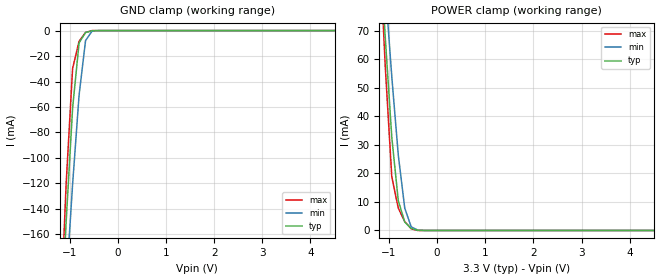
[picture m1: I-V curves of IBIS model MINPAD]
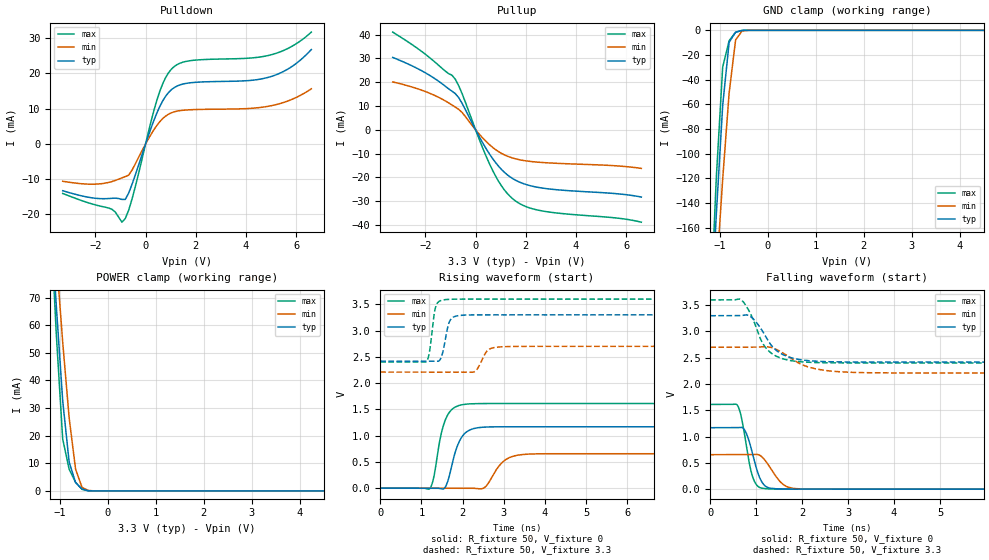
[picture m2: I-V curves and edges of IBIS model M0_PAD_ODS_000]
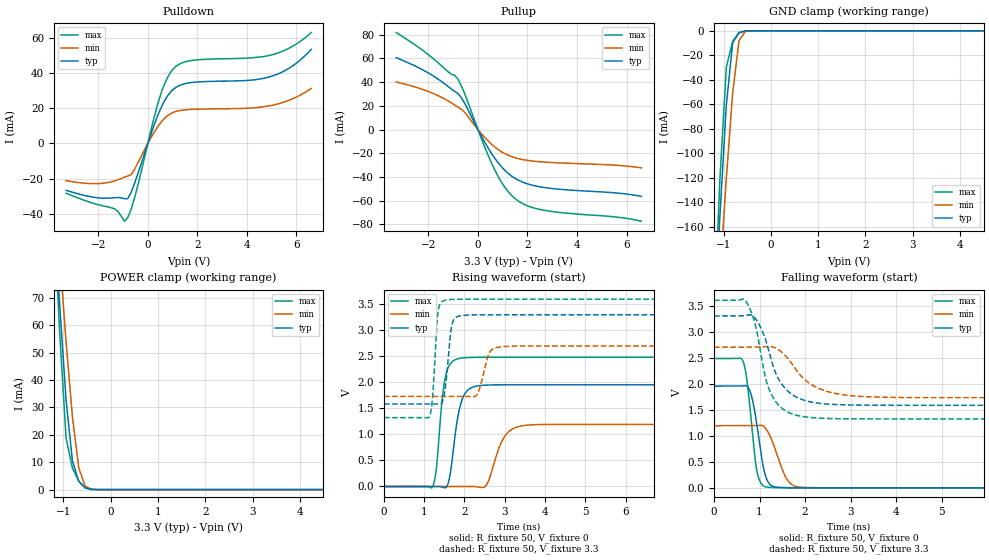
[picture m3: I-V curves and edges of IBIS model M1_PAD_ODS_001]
|   Microsemi Corporation
|   SmartFusion2 Automotive IBIS Model
[IBIS ver]   5.0
[File name]   as30208cg_33v_rev1p1.ibs
[File Rev]   1.1
[Date]   Wed Apr 02 2025
[Source] Simulated Models ONLY.
   All data is based on Spice simulation. All performed at Microsemi Corporation.
   Please refer to the Microsemi website for future updates at www.microsemi.com
[Notes]  Microsemi SmartFusion2 IBIS models for automotive operating conditions
   for DDRIO IO Banks IO Configurations ONLY. Models uses a software default
   fixed codes except for DDR3/SSTL15 which will always require calibrated
   codes.
   Automotive Temperature Grade 2 (t2) models cover a temperature range from
   -40C to 125C.
   Please refer to msio_auto_t2.ibs for MSIO IO Banks IO Configurations.
   Please refer to msiod_auto_t2.ibs for MSIOD IO Banks IO Configurations.
   The package parasitics of various package types are given.
   Uncomment the appropriate package or refer to the .pkg for specific
   per pin parasitic data.
   There are warnings related to non-monotonic and Increasing/Decreasing Current.
   They are expected on 20 Ohms and 30 Ohms I/O ODT models in DDR3/SSTL15.
[Disclaimer] This information is for board design considerations.
   Simulation based V/I curves contained in this model file are
   considered preliminary until verified against bench
   measurements. Maximum currents may vary from part to part but
   should not exceed maximum I/V curves provided in this model file.
[Copyright]  (c) 2015, Microsemi Corporation, All Rights Reserved.
| IBIS MODEL CHECKLIST
| Microsemi is dedicated to releasing quality IBIS models to customers.
| The following items have been
| verified for this IBIS model before release:
| 1)  Checked IBIS model by the golden parser ibischk5 [Complete]
| 2)  Ensured no errors reported by golden parser
|   for the IBIS model [Complete]
| 3)  Defined Vinl and Vinh for recievers [Complete]
| 4)  Defined Standard Load and Vmeas values for drivers [Complete]
| 5)  Defined overshoots for drivers and recievers [NA]
| 6)  Validated Ramp Values[Complete]
| 7)  Defined V-T Tables for all output drivers [Complete]
| 8)  Validated [Diff Pins] []
| 9)  Verified Package Parasitics [Complete]
| 10) Defined Standard Load Parameters and Specifications
|   for waveforms [Complete]
| 11) Defined and Validate Pin mappings [Complete]
| 12) Verified Ccomp Value []
| 13) Visually Inspected I-V Curves and V-T Tables  [Complete]
| 14) Presented Typ/Min/Max Values in the correct order for
|   all tables and parameters [Complete]
| 15) Simulated all output models with standard load and
|   switching through Vmeas [Complete]
| 16) Simulated all reciever models  [Complete]
| 17) Validated Models selectors. []
| 18) Visually inspected Spice and IBIS correlation for
|   a) Typical VT Curves [Complete]
|   b) Minimum VT Curves [Complete]
|   c) Maximum VT Curves [Complete]
| 19) Visually inspected Silicon and IBIS correlation
|   a) Typical IV Pull UP/ Pull Down Curves []
|   b) Minimum IV Pull UP/ Pull Down Curves []
|   c) Maximum IV Pull UP/ Pull Down Curves []
|   Component SmartFusion2
[Component]   SmartFusion2 W MRAM
[Manufacturer]   Avalanche Technology
[Package]
|  Design die-package: BGA
| variable   typ   min   max
R_pkg   0.72029   0.51528   1.0002
L_pkg   5.797e-9   4.155e-9   8.073e-9
C_pkg   1.116e-12   7.907e-13   1.753e-12
|Pin and Model info
[Pin]  signal_name  model_name   R_pin   L_pin   C_pin
L9   CS1#   MINPAD   0.4340		15.2000E-9		1.2600E-12
J10   CS2#   MINPAD   0.3800		13.5000E-9		1.0400E-12
K9   CLK1   MINPAD   0.4300		12.7000E-9		0.9790E-12
K8   CLK2   MINPAD   0.4480		14.6000E-9		1.1600E-12
M10   IO_0   MIOPAD   0.4010		12.4000E-9		1.2500E-12
M9   IO_1   MIOPAD   0.4050		14.2000E-9		1.1100E-12
L11   IO_2   MIOPAD   0.3780		11.8000E-9		1.2000E-12
M11   IO_3   MIOPAD   0.3700		11.8000E-9		1.2600E-12
M12   IO_4   MIOPAD   0.3710		11.1000E-9		1.1000E-12
N10   IO_5   MIOPAD   0.4050		13.8000E-9		1.1600E-12
N9   IO_6   MIOPAD   0.3830		15.2000E-9		1.0900E-12
N8   IO_7   MIOPAD   0.4480		16.4000E-9		1.0800E-12
J14   HTBSEL   MINPAD   0.1380		6.1700E-9		0.6060E-12
H14   HBP_2   MINPAD   0.1470		6.3900E-9		1.0000E-12
G13   HBP_1   MINPAD   0.1910		8.5000E-9		1.1500E-12
G12   HBP_0   MINPAD   0.2050		8.6800E-9		1.4200E-12
J11   RESET#   MINPAD   0.3410		14.1000E-9		1.6300E-12
J12   INT1#   MIOPAD   0.3080		12.5000E-9		1.2100E-12
K10   INT2#   MIOPAD   0.2120		10.3000E-9		0.8230E-12
M7   VSSIO   GND   NA   NA   NA
H8   VSSIO   GND   NA   NA   NA
L8   VSSIO   GND   NA   NA   NA
P10   VSSIO   GND   NA   NA   NA
H12   VSSIO   GND   NA   NA   NA
N12   VSSIO   GND   NA   NA   NA
P12   VSSIO   GND   NA   NA   NA
H13   VSSIO   GND   NA   NA   NA
N13   VSSIO   GND   NA   NA   NA
A3   VSS   GND   NA   NA   NA
B3   VSS   GND   NA   NA   NA
W3   VSS   GND   NA   NA   NA
Y3   VSS   GND   NA   NA   NA
A4   VSS   GND   NA   NA   NA
Y4   VSS   GND   NA   NA   NA
F5   VSS   GND   NA   NA   NA
G5   VSS   GND   NA   NA   NA
P5   VSS   GND   NA   NA   NA
R5   VSS   GND   NA   NA   NA
F6   VSS   GND   NA   NA   NA
H6   VSS   GND   NA   NA   NA
J6   VSS   GND   NA   NA   NA
L6   VSS   GND   NA   NA   NA
N6   VSS   GND   NA   NA   NA
R6   VSS   GND   NA   NA   NA
L7   VSS   GND   NA   NA   NA
N7   VSS   GND   NA   NA   NA
G8   VSS   GND   NA   NA   NA
P8   VSS   GND   NA   NA   NA
G10   VSS   GND   NA   NA   NA
H10   VSS   GND   NA   NA   NA
L12   VSS   GND   NA   NA   NA
L13   VSS   GND   NA   NA   NA
P13   VSS   GND   NA   NA   NA
F14   VSS   GND   NA   NA   NA
L14   VSS   GND   NA   NA   NA
N14   VSS   GND   NA   NA   NA
R14   VSS   GND   NA   NA   NA
F15   VSS   GND   NA   NA   NA
G15   VSS   GND   NA   NA   NA
P15   VSS   GND   NA   NA   NA
R15   VSS   GND   NA   NA   NA
A16   VSS   GND   NA   NA   NA
Y16   VSS   GND   NA   NA   NA
A17   VSS   GND   NA   NA   NA
B17   VSS   GND   NA   NA   NA
W17   VSS   GND   NA   NA   NA
Y17   VSS   GND   NA   NA   NA
G6   VCCIO   POWER   NA   NA   NA
P6   VCCIO   POWER   NA   NA   NA
G7   VCCIO   POWER   NA   NA   NA
J7   VCCIO   POWER   NA   NA   NA
P7   VCCIO   POWER   NA   NA   NA
M8   VCCIO   POWER   NA   NA   NA
H9   VCCIO   POWER   NA   NA   NA
H11   VCCIO   POWER   NA   NA   NA
N11   VCCIO   POWER   NA   NA   NA
J13   VCCIO   POWER   NA   NA   NA
M13   VCCIO   POWER   NA   NA   NA
G14   VCCIO   POWER   NA   NA   NA
P14   VCCIO   POWER   NA   NA   NA
K6   VCC   POWER   NA   NA   NA
M6   VCC   POWER   NA   NA   NA
K7   VCC   POWER   NA   NA   NA
G9   VCC   POWER   NA   NA   NA
P9   VCC   POWER   NA   NA   NA
G11   VCC   POWER   NA   NA   NA
K11   VCC   POWER   NA   NA   NA
P11   VCC   POWER   NA   NA   NA
K13   VCC   POWER   NA   NA   NA
K14   VCC   POWER   NA   NA   NA
M14   VCC   POWER   NA   NA   NA
K12   VDD   POWER   NA   NA   NA
| END PIN INFO
| IOPAD
[Model Selector] MIOPAD
| Model Description
M0_PAD_ODS_000   ODS_000
M1_PAD_ODS_001   ODS_001
M2_PAD_ODS_010   ODS_010
M3_PAD_ODS_011   ODS_011
M4_PAD_ODS_100   ODS_100
M5_PAD_ODS_101   ODS_101
M6_PAD_ODS_110   ODS_110
M7_PAD_ODS_111   ODS_111
| Models and submodels in the file (9): MINPAD (Input), M0_PAD_ODS_000 (I/O), M1_PAD_ODS_001 (I/O), M2_PAD_ODS_010 (I/O), M3_PAD_ODS_011 (I/O), M4_PAD_ODS_100 (I/O), M5_PAD_ODS_101 (I/O), M6_PAD_ODS_110 (I/O), M7_PAD_ODS_111 (I/O)
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[Model] MINPAD
Model_type Input
Enable   Active-High
Vinl  =  0.8
Vinh  =  2.2
| Capacitance  typ   min   max
C_comp   1.514821e-12   1.418868e-12   1.647023e-12
| Variables   typ   min   max
[GND Clamp Reference]   0   0   0
[POWER Clamp Reference]   3.3   2.7   3.6
[Pulldown Reference]   0   0   0
[Pullup Reference]   3.3   2.7   3.6
[Temperature Range]   25   125   -40
[Voltage Range]   3.3   2.7   3.6
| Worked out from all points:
|   GND clamp passes 1 mA (typ) near -0.62 V on its own axis
|   POWER clamp passes 1 mA (typ) near -0.56 V on its own axis
[GND Clamp]
| Voltage   I(typ)   I(min)   I(max)
-3.3V     -1.961A    -1.697A    -2.357A
-1.21V    -250.7mA   -283.7mA   -242.5mA
-1.076V   -150.6mA   -200.1mA   -120.6mA
-941.4mV  -60.83mA   -120.8mA   -29.75mA
-806.9mV  -9.646mA   -50.71mA   -8.435mA
-672.4mV  -1.585mA   -7.866mA   -1.457mA
-537.9mV  -71.75uA   -504.3uA   -18.73uA
-403.4mV  -593.9nA   -18.57uA   -37.22nA
6.6V      0A         0A         0A
[POWER Clamp]
| Voltage   I(typ)   I(min)   I(max)
-3.3V     772.3mA    673.3mA    930.5mA
-1.21V    105.9mA    117.6mA    104.6mA
-1.076V   67.34mA    85.06mA    57.16mA
-941.4mV  32.71mA    53.93mA    18.82mA
-806.9mV  10.48mA    26.53mA    7.848mA
-672.4mV  2.975mA    7.856mA    3.108mA
-537.9mV  710.9uA    1.248mA    573.1uA
-403.4mV  60.69uA    160.8uA    9.187uA
-269mV    142.4nA    6.118uA    23.26nA
6.6V      0A         0A         0A
[Model] M0_PAD_ODS_000
Model_type I/O
Enable   Active-High
Vinl  =  0.8
Vinh  =  2.2
Vmeas =  1.65
Cref  =  30e-12
| Capacitance  typ   min   max
C_comp   1.518749e-12   1.424706e-12   1.652746e-12
| Variables   typ   min   max
[GND Clamp Reference]   0   0   0
[POWER Clamp Reference]   3.3   2.7   3.6
[Pulldown Reference]   0   0   0
[Pullup Reference]   3.3   2.7   3.6
[Temperature Range]   25   125   -40
[Voltage Range]   3.3   2.7   3.6
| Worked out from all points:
|   slope of the pulldown table from 0 to 0.495 V, typ, clamps not added: 52.1 ohm
|   slope of the pullup table from 0 to 0.495 V, typ, clamps not added: 53.8 ohm
|   GND clamp passes 1 mA (typ) near -0.62 V on its own axis
|   POWER clamp passes 1 mA (typ) near -0.56 V on its own axis
|   falling waveform, R_fixture 50, V_fixture 0: 20-80 % time 230ps typ, 320ps min, 198ps max; typ from 1.17 V to 0 V
|   falling waveform, R_fixture 50, V_fixture 3.3: 20-80 % time 464ps typ, 644ps min, 396ps max; typ from 3.3 V to 2.42 V
|   rising waveform, R_fixture 50, V_fixture 0: 20-80 % time 273ps typ, 362ps min, 248ps max; typ from 0 V to 1.17 V
|   rising waveform, R_fixture 50, V_fixture 3.3: 20-80 % time 138ps typ, 198ps min, 114ps max; typ from 2.42 V to 3.3 V
[GND Clamp]
| Voltage   I(typ)   I(min)   I(max)
-3.3V     -1.961A    -1.697A    -2.357A
-1.21V    -250.7mA   -283.7mA   -242.5mA
-1.076V   -150.6mA   -200.1mA   -120.7mA
-941.4mV  -60.83mA   -120.8mA   -29.76mA
-806.9mV  -9.649mA   -50.71mA   -8.442mA
-672.4mV  -1.587mA   -7.866mA   -1.46mA
-537.9mV  -71.93uA   -504.3uA   -18.83uA
-403.4mV  -595.6nA   -18.58uA   -37.45nA
6.6V      0A         0A         0A
[POWER Clamp]
| Voltage   I(typ)   I(min)   I(max)
-3.3V     772.3mA    673.3mA    930.5mA
-1.21V    105.9mA    117.6mA    104.6mA
-1.076V   67.34mA    85.06mA    57.16mA
-941.4mV  32.71mA    53.93mA    18.82mA
-806.9mV  10.48mA    26.53mA    7.848mA
-672.4mV  2.975mA    7.856mA    3.108mA
-537.9mV  710.9uA    1.248mA    573.1uA
-403.4mV  60.69uA    160.8uA    9.187uA
-269mV    142.4nA    6.118uA    23.26nA
6.6V      0A         0A         0A
[Pulldown]
| Voltage   I(typ)   I(min)   I(max)
-3.3V     -13.26mA   -10.58mA   -14.05mA
-1.345V   -15.42mA   -10.67mA   -18.51mA
-941.4mV  -15.74mA   -9.611mA   -22.19mA
-806.9mV  -15.73mA   -9.263mA   -21.14mA
-537.9mV  -11.42mA   -7.417mA   -15.59mA
455.2mV   8.881mA    5.308mA    12.55mA
682.8mV   12.23mA    7.205mA    17.1mA
1.024V    15.38mA    8.837mA    21.2mA
1.821V    17.39mA    9.724mA    23.68mA
4.914V    18.96mA    10.73mA    25.16mA
5.783V    21.77mA    12.53mA    27.53mA
6.6V      26.8mA     15.66mA    31.75mA
[Pullup]
| Voltage   I(typ)   I(min)   I(max)
-3.3V     30.44mA    20.14mA    41.1mA
-1.883V   23.26mA    15.61mA    30.81mA
-806.9mV  15.23mA    9.539mA    21.27mA
-537.9mV  11.14mA    7.294mA    15.26mA
227.6mV   -4.448mA   -2.796mA   -6.209mA
682.8mV   -12.17mA   -7.42mA    -17.15mA
1.138V    -17.78mA   -10.49mA   -25.16mA
1.593V    -21.21mA   -12.21mA   -29.96mA
2.048V    -23.14mA   -13.13mA   -32.47mA
2.731V    -24.61mA   -13.8mA    -34.27mA
5.659V    -26.92mA   -15.2mA    -37.16mA
6.6V      -28.29mA   -16.23mA   -38.86mA
[Ramp]
dV/dt_r   0.701574/0.273396n  0.393696/0.362182n  0.967082/0.24767n
dV/dt_f   0.529393/0.463707n  0.294233/0.644316n  0.719379/0.396117n
R_load = 50
[Falling Waveform]
R_fixture = 50
V_fixture = 0
V_fixture_min = 0
V_fixture_max = 0
| Time   V(typ)   V(min)   V(max)
0s        1.169V     656.2mV    1.612V
592.6ps   1.17V      656.6mV    1.594V
662.7ps   1.175V     656.6mV    1.423V
757.8ps   1.11V      656.7mV    979.6mV
920.8ps   673.8mV    658.3mV    236.4mV
1.068ns   233.8mV    649.1mV    35.66mV
1.221ns   45.34mV    516.2mV    8.708mV
1.592ns   3.21mV     87.01mV    1.102mV
2.018ns   581.9uV    4.7mV      706uV
21.88ns   211nV      -2.279uV   3.818uV
[Falling Waveform]
R_fixture = 50
V_fixture = 3.3
V_fixture_min = 2.7
V_fixture_max = 3.6
| Time   V(typ)   V(min)   V(max)
0s        3.3V       2.7V       3.6V
662.6ps   3.302V     2.701V     3.609V
894.9ps   3.273V     2.701V     3.302V
1.117ns   3.036V     2.709V     2.815V
1.233ns   2.866V     2.709V     2.664V
1.51ns    2.594V     2.628V     2.502V
2.006ns   2.457V     2.366V     2.42V
2.5ns     2.427V     2.259V     2.405V
3.502ns   2.418V     2.214V     2.401V
21.88ns   2.418V     2.21V      2.401V
[Rising Waveform]
R_fixture = 50
V_fixture = 0
V_fixture_min = 0
V_fixture_max = 0
| Time   V(typ)   V(min)   V(max)
0s        11.89nV    88.47nV    -73.19nV
1.207ns   -862.4uV   -520.5uV   -4.427mV
1.285ns   -918.3uV   -554.2uV   157.9mV
1.593ns   39.36mV    -686.9uV   1.324V
1.858ns   773.7mV    -801.1uV   1.558V
2.069ns   1.055V     -892.4uV   1.599V
2.519ns   1.162V     5.17mV     1.611V
2.991ns   1.169V     510.2mV    1.611V
3.605ns   1.169V     648.6mV    1.611V
21.88ns   1.169V     656.2mV    1.612V
[Rising Waveform]
R_fixture = 50
V_fixture = 3.3
V_fixture_min = 2.7
V_fixture_max = 3.6
| Time   V(typ)   V(min)   V(max)
0s        2.418V     2.21V      2.401V
1.115ns   2.419V     2.21V      2.406V
1.19ns    2.419V     2.21V      2.571V
1.354ns   2.418V     2.21V      3.473V
1.494ns   2.522V     2.21V      3.578V
1.647ns   3.091V     2.21V      3.594V
2.284ns   3.299V     2.216V     3.599V
2.637ns   3.299V     2.641V     3.599V
3.102ns   3.299V     2.696V     3.599V
21.88ns   3.3V       2.7V       3.6V
[Model] M1_PAD_ODS_001
Model_type I/O
Enable   Active-High
Vinl  =  0.8
Vinh  =  2.2
Vmeas =  1.65
Cref  =  30e-12
| Capacitance  typ   min   max
C_comp   1.518749e-12   1.424706e-12   1.652746e-12
| Variables   typ   min   max
[GND Clamp Reference]   0   0   0
[POWER Clamp Reference]   3.3   2.7   3.6
[Pulldown Reference]   0   0   0
[Pullup Reference]   3.3   2.7   3.6
[Temperature Range]   25   125   -40
[Voltage Range]   3.3   2.7   3.6
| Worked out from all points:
|   slope of the pulldown table from 0 to 0.495 V, typ, clamps not added: 26.1 ohm
|   slope of the pullup table from 0 to 0.495 V, typ, clamps not added: 27 ohm
|   GND clamp passes 1 mA (typ) near -0.62 V on its own axis
|   POWER clamp passes 1 mA (typ) near -0.56 V on its own axis
|   falling waveform, R_fixture 50, V_fixture 0: 20-80 % time 211ps typ, 305ps min, 176ps max; typ from 1.95 V to 0 V
|   falling waveform, R_fixture 50, V_fixture 3.3: 20-80 % time 457ps typ, 660ps min, 366ps max; typ from 3.3 V to 1.58 V
|   rising waveform, R_fixture 50, V_fixture 0: 20-80 % time 225ps typ, 335ps min, 176ps max; typ from 0 V to 1.95 V
|   rising waveform, R_fixture 50, V_fixture 3.3: 20-80 % time 129ps typ, 193ps min, 104ps max; typ from 1.58 V to 3.3 V
[GND Clamp]
| Voltage   I(typ)   I(min)   I(max)
-3.3V     -1.961A    -1.697A    -2.357A
-1.21V    -250.7mA   -283.7mA   -242.5mA
-1.076V   -150.6mA   -200.1mA   -120.7mA
-941.4mV  -60.83mA   -120.8mA   -29.76mA
-806.9mV  -9.649mA   -50.71mA   -8.442mA
-672.4mV  -1.587mA   -7.866mA   -1.46mA
-537.9mV  -71.93uA   -504.3uA   -18.83uA
-403.4mV  -595.6nA   -18.58uA   -37.45nA
6.6V      0A         0A         0A
[POWER Clamp]
| Voltage   I(typ)   I(min)   I(max)
-3.3V     772.3mA    673.3mA    930.5mA
-1.21V    105.9mA    117.6mA    104.6mA
-1.076V   67.34mA    85.06mA    57.16mA
-941.4mV  32.71mA    53.93mA    18.82mA
-806.9mV  10.48mA    26.53mA    7.848mA
-672.4mV  2.975mA    7.856mA    3.108mA
-537.9mV  710.9uA    1.248mA    573.1uA
-403.4mV  60.69uA    160.8uA    9.187uA
-269mV    142.4nA    6.118uA    23.26nA
6.6V      0A         0A         0A
[Pulldown]
| Voltage   I(typ)   I(min)   I(max)
-3.3V     -26.68mA   -21.22mA   -28.37mA
-1.345V   -30.89mA   -21.35mA   -37.2mA
-941.4mV  -31.46mA   -19.19mA   -44.32mA
-806.9mV  -31.44mA   -18.5mA    -42.21mA
-537.9mV  -22.81mA   -14.83mA   -31.1mA
455.2mV   17.74mA    10.61mA    25.04mA
682.8mV   24.44mA    14.41mA    34.16mA
1.024V    30.75mA    17.67mA    42.38mA
1.821V    34.78mA    19.45mA    47.35mA
4.914V    37.93mA    21.47mA    50.14mA
5.783V    43.54mA    25.06mA    54.82mA
6.6V      53.61mA    31.34mA    63.15mA
[Pullup]
| Voltage   I(typ)   I(min)   I(max)
-3.3V     60.61mA    40.12mA    81.78mA
-1.883V   46.22mA    31.07mA    61.18mA
-806.9mV  30.34mA    18.97mA    42.44mA
-537.9mV  22.21mA    14.55mA    30.44mA
227.6mV   -8.868mA   -5.574mA   -12.38mA
682.8mV   -24.26mA   -14.79mA   -34.2mA
1.138V    -35.44mA   -20.91mA   -50.18mA
1.593V    -42.28mA   -24.34mA   -59.75mA
2.048V    -46.13mA   -26.16mA   -64.77mA
2.731V    -49.08mA   -27.51mA   -68.35mA
5.659V    -53.66mA   -30.27mA   -74.01mA
6.6V      -56.41mA   -32.34mA   -77.42mA
[Ramp]
dV/dt_r   1.17185/0.224543n  0.715782/0.335331n  1.48949/0.176355n
dV/dt_f   1.02933/0.457397n  0.581576/0.659988n  1.3662/0.365774n
R_load = 50
[Falling Waveform]
R_fixture = 50
V_fixture = 0
V_fixture_min = 0
V_fixture_max = 0
| Time   V(typ)   V(min)   V(max)
0s        1.953V     1.193V     2.482V
635.9ps   1.956V     1.193V     2.431V
704.7ps   1.96V      1.193V     2.173V
796.3ps   1.84V      1.193V     1.481V
940.8ps   1.211V     1.196V     323.6mV
1.07ns    457mV      1.192V     48.18mV
1.162ns   158.1mV    1.107V     14.87mV
1.596ns   3.876mV    172.7mV    1.351mV
1.955ns   1.021mV    9.401mV    393uV
21.88ns   -91.88nV   -824.1nV   -402.1nV
[Falling Waveform]
R_fixture = 50
V_fixture = 3.3
V_fixture_min = 2.7
V_fixture_max = 3.6
| Time   V(typ)   V(min)   V(max)
0s        3.3V       2.7V       3.6V
680.8ps   3.304V     2.7V       3.601V
875.3ps   3.282V     2.701V     3.232V
992.1ps   3.135V     2.701V     2.762V
1.133ns   2.84V      2.714V     2.105V
1.288ns   2.362V     2.705V     1.747V
1.59ns    1.883V     2.517V     1.468V
2.081ns   1.658V     2.016V     1.353V
3.936ns   1.585V     1.736V     1.323V
21.88ns   1.584V     1.731V     1.323V
[Rising Waveform]
R_fixture = 50
V_fixture = 0
V_fixture_min = 0
V_fixture_max = 0
| Time   V(typ)   V(min)   V(max)
0s        8.206nV    63.6nV     -79.24nV
1.21ns    786.9uV    36.26uV    -2.765mV
1.297ns   843.1uV    38.84uV    308mV
1.529ns   -24.63mV   45.8uV     2.116V
1.633ns   186.3mV    48.92uV    2.341V
1.918ns   1.614V     57.42uV    2.467V
2.501ns   1.946V     -8.282mV   2.482V
3.016ns   1.953V     981.7mV    2.482V
3.576ns   1.953V     1.179V     2.482V
21.88ns   1.953V     1.193V     2.482V
[Rising Waveform]
R_fixture = 50
V_fixture = 3.3
V_fixture_min = 2.7
V_fixture_max = 3.6
| Time   V(typ)   V(min)   V(max)
0s        1.584V     1.731V     1.323V
1.129ns   1.585V     1.731V     1.34V
1.203ns   1.585V     1.731V     1.679V
1.346ns   1.586V     1.731V     3.368V
1.476ns   1.69V      1.731V     3.568V
1.581ns   2.324V     1.732V     3.588V
1.708ns   3.159V     1.732V     3.595V
2.034ns   3.293V     1.732V     3.599V
2.983ns   3.299V     2.689V     3.599V
21.88ns   3.3V       2.7V       3.6V
